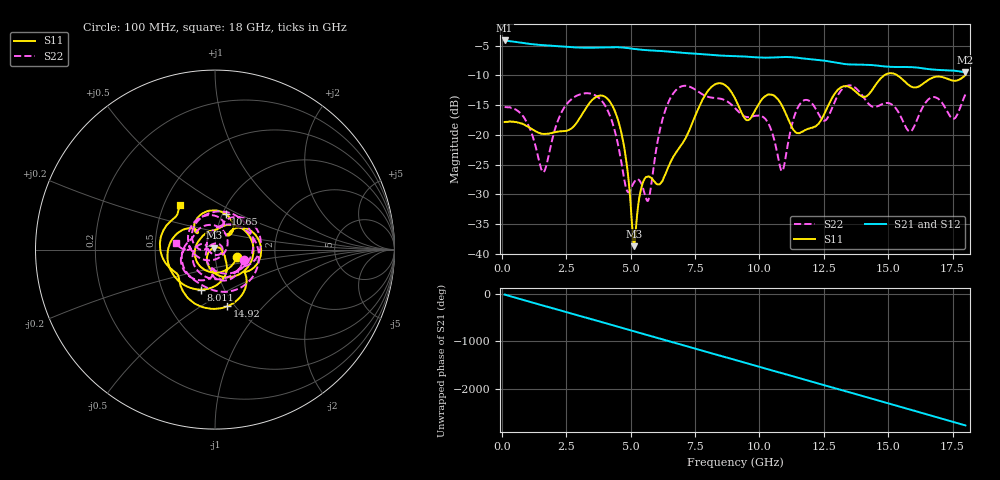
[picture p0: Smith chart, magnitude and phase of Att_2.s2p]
#  HZ  S  DB  R  50.00
! Rohde & Schwarz Vector Network Analyzer
! Rohde-Schwarz,ZNB40-4Port,1311601084101679,3.45
! Created: UTC 4/25/2025, 8:43:06 AM
! freq[Hz]  db:S11  ang:S11  db:S21  ang:S21  db:S12  ang:S12  db:S22  ang:S22
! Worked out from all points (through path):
!   1750 points, 100 MHz to 18 GHz, reference 50 ohm
!   highest |S21| = -4.12 dB at 100 MHz (marker M1); lowest = -9.5 dB at 18 GHz (marker M2)
!   group delay of S21, straight-line fit = 428 ps
!   lowest |S11| = -38.7 dB at 5.125 GHz (marker M3), VSWR 1.02, Z = 49.6 + j1.11 ohm
!   |S11| at or under -10 dB: start of sweep to 14.84 GHz; 15.36 GHz to 17.99 GHz (2.629 GHz wide, 15.8 % of centre)
!   |S22| runs from -31.1 to -11.7 dB; largest |S21 - S12| = 0.00077
!   S11 on the Smith chart (normalised r, x): 100 MHz: 1.27, -0.11; 8.011 GHz: 0.78, -0.37; 10.65 GHz: 1.04, +0.43; 14.92 GHz: 0.92, -0.65; 18 GHz: 0.60, +0.34
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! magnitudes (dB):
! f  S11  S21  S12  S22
! 100 MHz  -17.8  -4.1  -4.1  -15.3
! 898.3 MHz  -18.4  -4.6  -4.6  -17.4
! 1.604 GHz  -19.8  -4.9  -4.9  -26.3
! 2.3 GHz  -19.4  -5.1  -5.1  -16.3
! 3.088 GHz  -16.7  -5.3  -5.3  -13.1
! 4.358 GHz  -15.7  -5.2  -5.2  -18.9
! 4.777 GHz  -22.9  -5.4  -5.4  -28.1
! 5.125 GHz  -38.7  -5.5  -5.5  -28.0
! 5.678 GHz  -26.9  -5.8  -5.8  -31.0
! 6.067 GHz  -28.3  -5.9  -5.9  -20.5
! 6.814 GHz  -22.6  -6.1  -6.1  -12.2
! 8.011 GHz  -12.5  -6.5  -6.5  -13.6
! 9.055 GHz  -13.9  -6.8  -6.8  -15.5
! 9.536 GHz  -17.5  -6.9  -6.9  -17.0
! 10.65 GHz  -13.7  -7.0  -7.0  -22.2
! 10.9 GHz  -15.3  -6.9  -6.9  -26.0
! 11.46 GHz  -19.7  -7.0  -7.0  -15.7
! 12.04 GHz  -18.8  -7.3  -7.3  -14.7
! 14.92 GHz  -9.8  -8.5  -8.5  -14.6
! 15.02 GHz  -9.7  -8.5  -8.5  -14.7
! 15.85 GHz  -11.8  -8.6  -8.6  -19.4
! 18 GHz  -10.0  -9.5  -9.5  -13.2
